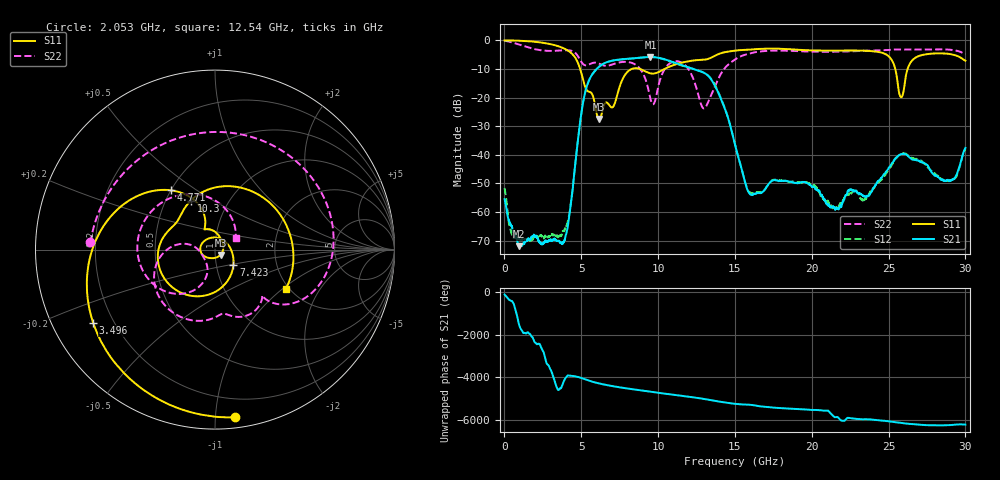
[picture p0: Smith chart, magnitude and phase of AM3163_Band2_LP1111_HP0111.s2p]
!Agilent Technologies,E8364B,MY43040894,A.07.50.67
!Agilent E8364B: A.07.50.67
!Date: Thursday, August 20, 2020 12:07:57
!Correction: S11(Full 2 Port(1,2))
!S21(Full 2 Port(1,2))
!S12(Full 2 Port(1,2))
!S22(Full 2 Port(1,2))
!S2P File: Measurements: S11, S21, S12, S22:
# Hz S  dB  R 50
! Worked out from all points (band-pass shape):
!   3201 points, 10 MHz to 30 GHz, reference 50 ohm
!   highest |S21| = -5.79 dB at 9.504 GHz (marker M1); lowest = -71.9 dB at 928.4 MHz (marker M2)
!   |S21| within 3 dB of the highest: 6.255 GHz to 11.62 GHz (5.365 GHz wide, 60 % of centre)
!   lowest |S11| = -27.4 dB at 6.167 GHz (marker M3), VSWR 1.09, Z = 53.1 - j3.1 ohm
!   |S11| at or under -10 dB: 4.926 GHz to 8.277 GHz (3.351 GHz wide, 50.8 % of centre); 8.821 GHz to 10.41 GHz (1.593 GHz wide, 16.6 % of centre); 25.44 GHz to 26.24 GHz (800.8 MHz wide, 3.1 % of centre)
!   |S22| runs from -23.8 to -0.2 dB; largest |S21 - S12| = 0.012
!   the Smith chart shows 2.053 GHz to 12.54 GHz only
!   S11 on the Smith chart (normalised r, x): 2.053 GHz: 0.07, -1.12; 3.496 GHz: 0.12, -0.27; 4.771 GHz: 0.50, +0.40; 7.423 GHz: 1.21, -0.21; 10.3 GHz: 0.67, +0.40; 12.54 GHz: 1.93, -1.06
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1e7  -0.02 -2.6  -55.51 -131.3  -51.58 -86.1  -0.16 -6.9
9.284438e8  -0.09 -37.1  -71.91 -39.1  -69.27 -1.8  -1.40 -88.8
2.053069e9  -0.53 -83.3  -68.36 119.6  -68.89 107.3  -3.16 176.6
3.496338e9  -2.02 -148.9  -70.16 87.6  -68.83 -77.4  -3.59 66.6
4.05865e9  -3.32 179.6  -66.46 -3.1  -64.45 29.3  -3.45 24.2
4.770912e9  -7.70 126.7  -35.37 -19.9  -35.37 -19.7  -5.42 -33.4
5.014581e9  -11.68 109.6  -25.08 -73.1  -25.12 -73.3  -7.59 -43.7
6.167322e9  -27.44 -43.4  -9.16 33.7  -9.20 33.5  -8.14 -72.8
7.423153e9  -17.47 -40.0  -6.71 -138.3  -6.78 -138.2  -7.77 -103.9
8.585266e9  -9.74 -162.2  -6.17 99.9  -6.17 100.1  -8.70 -157.3
9.503709e9  -11.52 148.8  -5.79 9.3  -5.78 9.1  -20.53 179.8
1.000979e10  -11.12 130.8  -6.06 -41.0  -6.09 -41.6  -16.13 -107.9
1.030032e10  -10.32 116.2  -6.40 -69.5  -6.50 -70.2  -11.31 -120.2
1.25402e10  -6.89 -28.9  -10.44 80.2  -10.39 81.5  -17.52 29.9
1.5005e10  -3.58 -132.5  -36.51 160.8  -36.40 159.9  -6.69 -112.2
1.599842e10  -3.21 -173.8  -53.80 118.2  -53.14 117.1  -4.52 -172.1
1.787279e10  -2.91 98.2  -49.09 -37.4  -48.96 -36.7  -3.57 92.0
2.000958e10  -3.50 -9.9  -51.12 -121.0  -50.48 -118.5  -3.94 -9.5
2.231506e10  -3.54 -100.0  -53.55 -130.8  -53.63 -138.9  -3.86 -93.8
2.500479e10  -5.54 157.6  -44.61 69.5  -45.23 68.6  -3.36 -167.7
2.582014e10  -19.85 171.7  -39.79 -7.1  -39.57 -7.2  -3.21 170.2
3e10  -7.11 51.8  -37.55 -87.1  -37.80 -87.6  -4.77 55.4
